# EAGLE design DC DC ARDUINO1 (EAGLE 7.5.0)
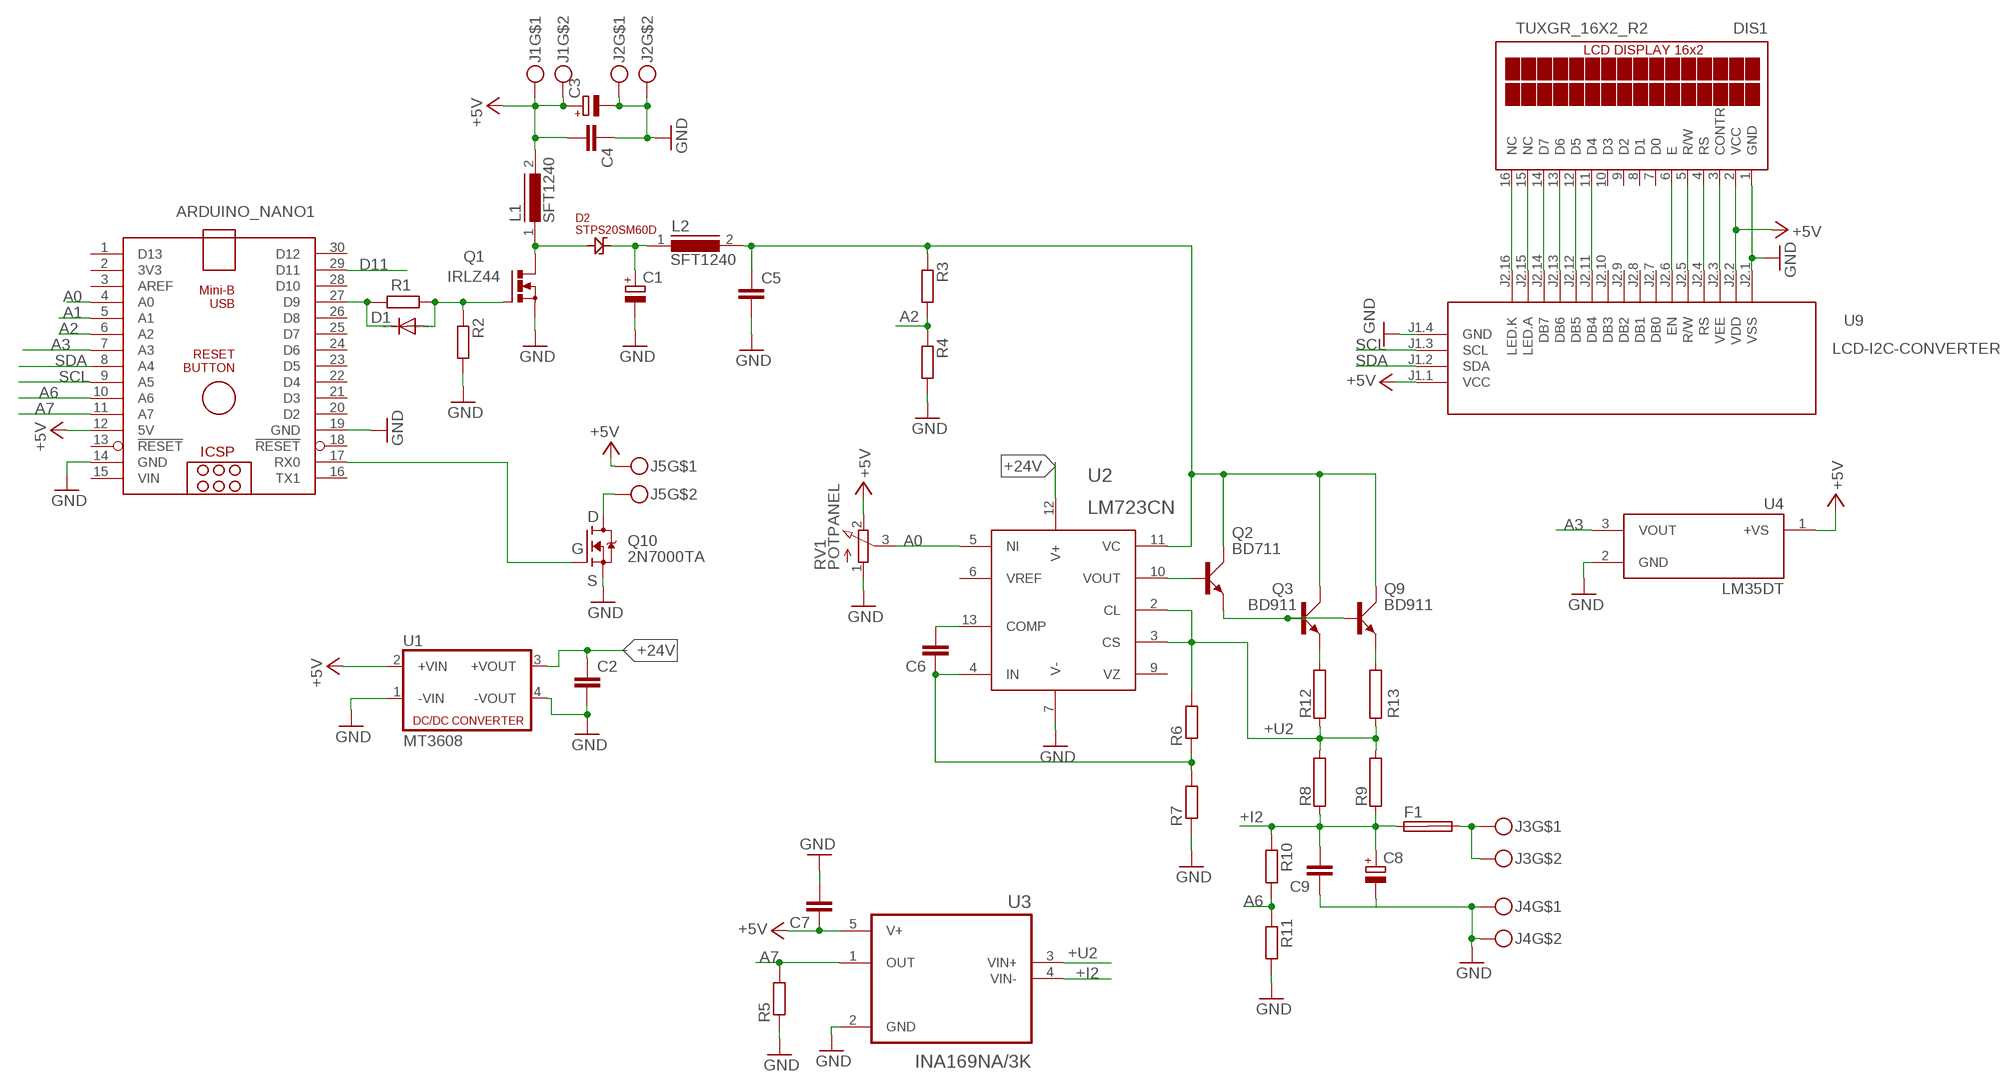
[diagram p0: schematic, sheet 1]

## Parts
ARDUINO_NANO1  ARDUINO_NANO  [ARDUINO_NANO]
C1  CPOL-EUE7.5-18  [E7,5-18]
C2  C-EU050-030X075  [C050-030X075]
C3  CPOL-EUE7.5-18  [E7,5-18]
C4  C-EU050-030X075  [C050-030X075]
C5  C-EU050-030X075  [C050-030X075]
C6  C-EU050-030X075  [C050-030X075]
C7  C-EU050-030X075  [C050-030X075]
C8  CPOL-EUE7.5-18  [E7,5-18]
C9  C-EU050-030X075  [C050-030X075]
D1  1N4148DO35-10  [DO35-10]
D2  STPS20SM60D  [TO-220-2]
DIS1  TUXGR_16X2_R2  [TUXGR_16X2_R2]
F1  SHK20L  [SHK20L]
J1  MKDSN1,5-2-5,08  [MKDSN1,5-2-5,08]
J2  MKDSN1,5-2-5,08  [MKDSN1,5-2-5,08]
J3  MKDSN1,5-2-5,08  [MKDSN1,5-2-5,08]
J4  MKDSN1,5-2-5,08  [MKDSN1,5-2-5,08]
J5  MKDSN1,5-2-5,08  [MKDSN1,5-2-5,08]
L1  SFT1240  [SFT1240]
L2  SFT1240  [SFT1240]
Q1  IRLZ44  IRF512  [TO220BV]
Q2  BD711  MJE3055  [TO220AV]
Q3  BD911  MJE3055  [TO220AV]
Q9  BD911  MJE3055  [TO220AV]
Q10  2N7000TA  [TO-92]
R1  R-EU_  [0204_6]
R2  R-EU_  [0204_6]
R3  R-EU_  [0204_6]
R4  R-EU_  [0204_6]
R5  R-EU_  [0204_6]
R6  R-EU_  [0204_6]
R7  R-EU_  [0204_6]
R8  RCA4050  [CA4050]
R9  RCA4050  [CA4050]
R10  R-EU_  [0204_6]
R11  R-EU_  [0204_6]
R12  RCA4050  [CA4050]
R13  RCA4050  [CA4050]
RV1  POTPANEL  [POTPANELP231]
U1  MT3608  [MT3608]
U2  LM723CN  [DIP14]
U3  INA169NA/3K  [SOT95P280X145-5N]
U4  LM35DT  [TO254P1016X457X1955-3]
U9  LCD-I2C-CONVERTER  [LCD-I2C-CONVERTER]

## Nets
+5V: ARDUINO_NANO1.12(5V) C3.+ C4.2 C7.1 DIS1.2(VCC) J1.1 J1.2 J5.1 L1.2 RV1.2(E) U1.2(+VIN) U3.5(V+) U4.1(+VS) U9.J1.1(VCC) U9.J2.2(VDD)
+24V: C2.1 U1.3(+VOUT) U2.12(V+)
+I2: C8.+ C9.2 F1.1A R8.1 R9.1 R10.1 U3.4(VIN-)
+U2: R6.2 R8.2 R9.2 R12.1 R13.1 U2.2(CL) U2.3(CS) U3.3(VIN+)
A0: ARDUINO_NANO1.4(A0) RV1.3(S) U2.5(NI)
A1: ARDUINO_NANO1.5(A1)
A2: ARDUINO_NANO1.6(A2) R3.2 R4.1
A3: ARDUINO_NANO1.7(A3) U4.3(VOUT)
A6: ARDUINO_NANO1.10(A6) R10.2 R11.1
A7: ARDUINO_NANO1.11(A7) R5.2 U3.1(OUT)
D11: ARDUINO_NANO1.29(D11)
GND: ARDUINO_NANO1.14(GND) ARDUINO_NANO1.19(GND) C1.- C2.2 C3.- C4.1 C5.2 C7.2 C8.- C9.1 DIS1.1(GND) J2.1 J2.2 J4.1 J4.2 Q1.S Q10.1(S) R2.2 R4.2 R5.1 R7.1 R11.2 RV1.1(A) U1.1(-VIN) U1.4(-VOUT) U2.7(V-) U3.2(GND) U4.2(GND) U9.J1.4(GND) U9.J2.1(VSS)
N$1: Q3.E R12.2
N$2: Q9.E R13.2
N$4: F1.2A J3.1 J3.2
N$5: ARDUINO_NANO1.17(RX0) Q10.2(G)
N$6: D1.A Q1.G R1.1 R2.1
N$7: ARDUINO_NANO1.27(D9) D1.C R1.2
N$8: D2.3(A) L1.1 Q1.D
N$9: J5.2 Q10.3(D)
N$10: C5.1 L2.2 Q2.C Q3.C Q9.C R3.1 U2.11(VC)
N$11: C1.+ D2.1(K) L2.1
N$23: C6.2 U2.13(COMP)
N$24: Q2.E Q3.B Q9.B
N$26: C6.1 R6.1 R7.2 U2.4(IN)
N$27: Q2.B U2.10(VOUT)
N$31: DIS1.3(CONTR) U9.J2.3(VEE)
N$32: DIS1.4(RS) U9.J2.4(RS)
N$33: DIS1.5(R/W) U9.J2.5(R/W)
N$34: DIS1.6(E) U9.J2.6(EN)
N$35: DIS1.14(D7) U9.J2.14(DB7)
N$36: DIS1.13(D6) U9.J2.13(DB6)
N$37: DIS1.12(D5) U9.J2.12(DB5)
N$38: DIS1.11(D4) U9.J2.11(DB4)
N$39: DIS1.16(NC) U9.J2.16(LED.K)
N$40: DIS1.15(NC) U9.J2.15(LED.A)
SCL: ARDUINO_NANO1.9(A5) U9.J1.3(SCL)
SDA: ARDUINO_NANO1.8(A4) U9.J1.2(SDA)
Unconnected: ARDUINO_NANO1.1(D13) ARDUINO_NANO1.2(3V3) ARDUINO_NANO1.3(AREF) ARDUINO_NANO1.13(!RESET) ARDUINO_NANO1.16(TX1) ARDUINO_NANO1.18(!RESET) ARDUINO_NANO1.20(D2) ARDUINO_NANO1.21(D3) ARDUINO_NANO1.22(D4) ARDUINO_NANO1.23(D5) ARDUINO_NANO1.24(D6) ARDUINO_NANO1.25(D7) ARDUINO_NANO1.26(D8) ARDUINO_NANO1.28(D10) ARDUINO_NANO1.30(D12) DIS1.7(D0) DIS1.8(D1) DIS1.9(D2) DIS1.10(D3) F1.1B F1.2B U2.6(VREF) U2.9(VZ) U9.J2.7(DB0) U9.J2.8(DB1) U9.J2.9(DB2) U9.J2.10(DB3)

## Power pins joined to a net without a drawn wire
VIN: ARDUINO_NANO1.15(VIN)

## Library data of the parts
ARDUINO_NANO1 = ArduinoNanoV30:ARDUINO_NANO: Arduino Nano V3.0 Overview: The Arduino Nano is a small, complete, and breadboard-friendly board based on the ATmega328 (Arduino Nano 3.x) or ATmega168 (Arduino Nano 2.x). It has more or less the same functionality of the Arduino Duemilanove, but in a different package. It lacks only a DC power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
C1 C3 C8 = rcl:CPOL-EU: POLARIZED CAPACITOR, European symbol
C2 C4-C7 C9 = rcl:C-EU: CAPACITOR, European symbol
D1 = diode:1N4148: DIODE
D2 = STPS20SM60D:STPS20SM60D: Diode Schottky 60V 20A Through Hole TO-220AC Check availability; AVAILABILITY: In Stock; CHECK_PRICES: https://www.snapeda.com/parts/STPS20SM60D/STMicroelectronics/view-part/?ref=eda; DESCRIPTION: Diode Schottky 60 V 20A Through Hole TO-220AC; MF: STMicroelectronics; MP: STPS20SM60D; PACKAGE: TO-220 STMicroelectronics; PRICE: None; PURCHASE-URL: https://www.snapeda.com/api/url_track_click_mouser/?unipart_id=727029&manufacturer=STMicroelectronics&part_name=STPS20SM60D&search_term=shottky diode 20a to-220; SNAPEDA_LINK: https://www.snapeda.com/parts/STPS20SM60D/STMicroelectronics/view-part/?ref=snap
DIS1 = display-lcd:TUXGR_16X2_R2: Tuxgraphics LCD display 16x2 characters reflective, without background light Source: tuxgr_12x2_r2.pdf; OC_FARNELL: unknown; OC_NEWARK: unknown
F1 = fuse:SHK20L: FUSE HOLDER 5 x 20 mm, SH contact, SHH1 Schukat, E1073 Buerklin; OC_FARNELL: unknown; OC_NEWARK: unknown
J1-J5 = con-phoenix-508:MKDSN1,5-2-5,08
L1 L2 = inductors:SFT1240: INDUCTOR
Q1 = transistor-power:IRF512: N-CHANNEL MOS FET
Q2 Q3 Q9 = transistor-power:MJE3055: NPN TRANSISTOR
Q10 = 2N7000TA:2N7000TA: http://www.mouser.com/ds/2/149/2N7000TA-347571.pdf Check availability; AVAILABILITY: In Stock; CHECK_PRICES: https://www.snapeda.com/parts/2N7000-TA/Onsemi/view-part/?ref=eda; DESCRIPTION: N-Channel 60 V 200mA (Tc) 400mW (Ta) Through Hole TO-92-3; MF: ON Semiconductor; MP: 2N7000-TA; PACKAGE: E-PKG AXIAL-LEADED-2 ON Semiconductor; PRICE: None; SNAPEDA_LINK: https://www.snapeda.com/parts/2N7000-TA/Onsemi/view-part/?ref=snap
R1-R7 R10 R11 = rcl:R-EU_: RESISTOR, European symbol
R8 R9 R12 R13 = resistor-power:R: Power Resitor; OC_FARNELL: unknown; OC_NEWARK: unknown
RV1 = pot:POTPANEL
U1 = dc-dc-converter:MT3608: DC DC Up Converter
U2 = v-reg:LM723CN: 150mA out, Voltage Regulator
U3 = INA169NA_3K:INA169NA/3K: Check availability; AVAILABILITY: In Stock; CHECK_PRICES: https://www.snapeda.com/parts/INA169NA/3K/Texas+Instruments/view-part/?ref=eda; DESCRIPTION: 2.7 to 60V, 440kHz Variable gain current sense amplifier; MF: Texas Instruments; MP: INA169NA/3K; PACKAGE: SOT-23-5 Texas Instruments; PRICE: None; PURCHASE-URL: https://pricing.snapeda.com/search?q=INA169NA/3K&ref=eda; SNAPEDA_LINK: https://www.snapeda.com/parts/INA169NA/3K/Texas+Instruments/view-part/?ref=snap
U4 = LM35DT-H:LM35DT: Check availability; AVAILABILITY: In Stock; CHECK_PRICES: https://www.snapeda.com/parts/LM35DT/Texas+Instruments/view-part/?ref=eda; DESCRIPTION: ±0.5°C 4V-30V, Temperature sensor with analog output 3-TO-220 0 to 100; MF: Texas Instruments; MP: LM35DT; PACKAGE: TO-220-3 Texas Instruments; PRICE: None; SNAPEDA_LINK: https://www.snapeda.com/parts/LM35DT/Texas+Instruments/view-part/?ref=snap
U9 = diy-modules:LCD-I2C-CONVERTER: I2C Bus to 4-Bit Parallel LCD Interface with LED backlight driver

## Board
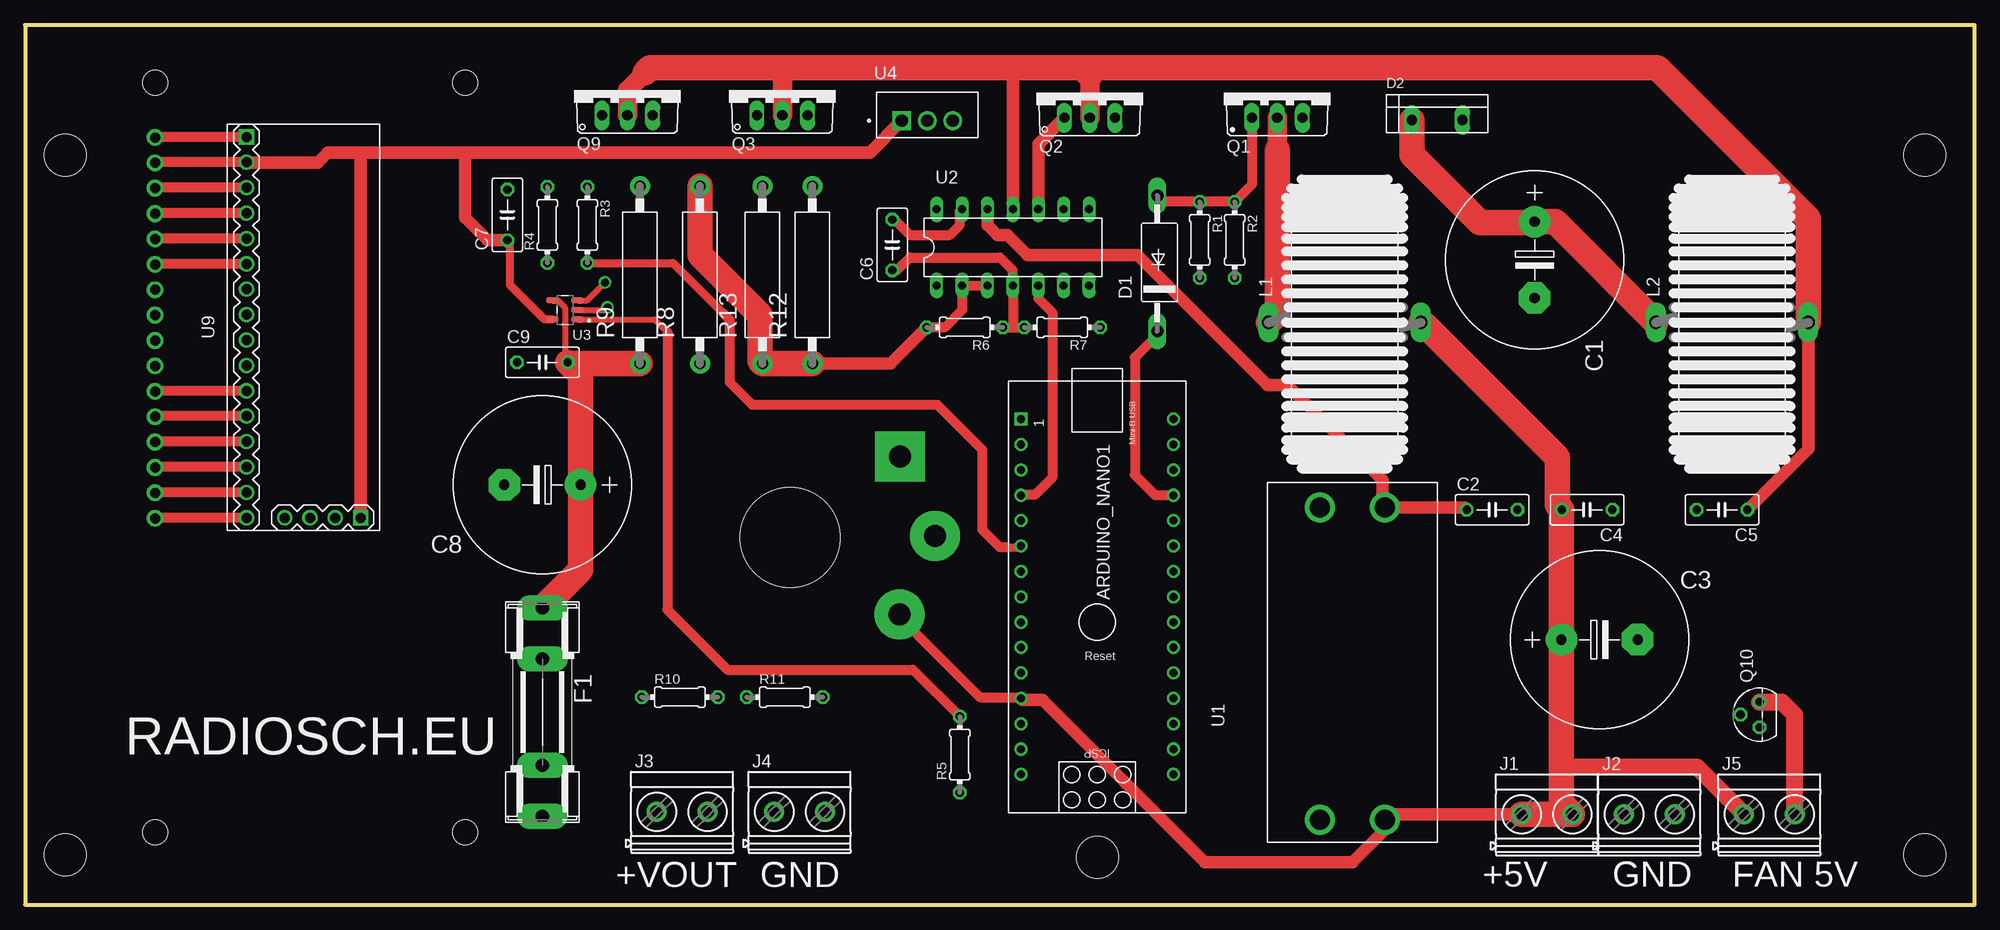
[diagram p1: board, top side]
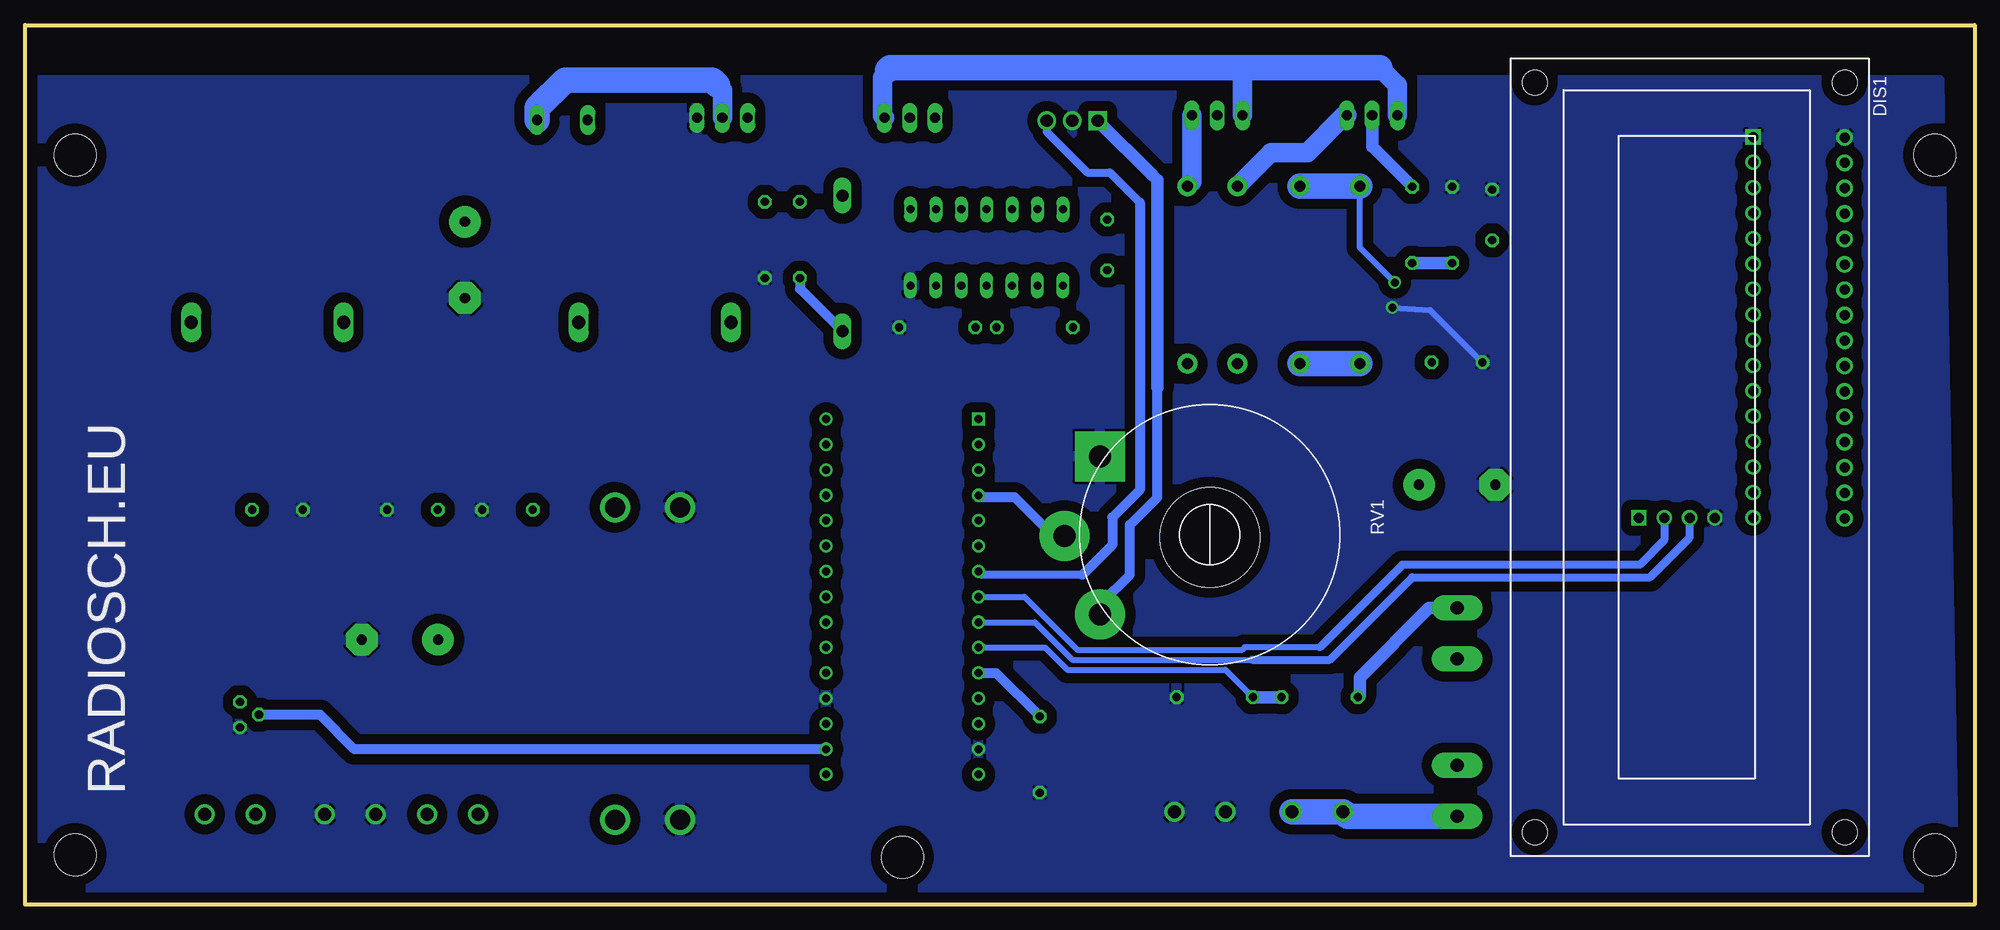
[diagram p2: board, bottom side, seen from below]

Size 195 x 88 mm. Coordinates in mm from the lower left corner, seen from the top.
Outline: 0,0 195,0 195,88 0,88 0,0
Copper layers (1*16): Top 0.035mm / dielectric 1.5mm / Bottom 0.035mm
Design rules "default": minimum track width 10mil, minimum drill 24mil, track to track 8mil, track to pad 8mil, pad to pad 8mil, via to via 8mil, smd to smd 8mil, copper to edge 40mil, drill to drill 8mil, minimum pad ring 10mil, minimum via ring 8mil, stop-mask expansion 4mil, vias tented up to drill 0mil, thermal gap 10mil
Holes 4.2 mm at 4,75 107.25,4.75 190,75 190,5 4,5
Holes 10 mm at 76.5,36.75

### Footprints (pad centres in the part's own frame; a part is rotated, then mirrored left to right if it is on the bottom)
ARDUINO_NANO = drill 0.8 square: 1 -20.32,-7.62 | drill 0.8: 2 -17.78,-7.62; 3 -15.24,-7.62; 4 -12.7,-7.62; 5 -10.16,-7.62; 6 -7.62,-7.62; 7 -5.08,-7.62; 8 -2.54,-7.62; 9 0,-7.62; 10 2.54,-7.62; 11 5.08,-7.62; 12 7.62,-7.62; 13 10.16,-7.62; 14 12.7,-7.62; 15 15.24,-7.62; 16 15.24,7.62; 17 12.7,7.62; 18 10.16,7.62; 19 7.62,7.62; 20 5.08,7.62; 21 2.54,7.62; 22 0,7.62; 23 -2.54,7.62; 24 -5.08,7.62; 25 -7.62,7.62; 26 -10.16,7.62; 27 -12.7,7.62; 28 -15.24,7.62; 29 -17.78,7.62; 30 -20.32,7.62
E7,5-18 = drill 1.016 pad 3.15: + -3.81,0 | drill 1.016 pad 3.15 octagon: - 3.81,0
C050-030X075 = drill 0.813 octagon: 1 -2.54,0; 2 2.54,0
DO35-10 = drill 1.2 long: A 8.18,0; C -5.38,0
TO-220-2 = drill 1.016 long: 1 -2.54,0; 3 2.54,0
TUXGR_16X2_R2 = drill 1 pad 1.676: 1 -32,15.5; 2 -29.46,15.5; 3 -26.92,15.5; 4 -24.38,15.5; 5 -21.84,15.5; 6 -19.3,15.5; 7 -16.76,15.5; 8 -14.22,15.5; 9 -11.68,15.5; 10 -9.14,15.5; 11 -6.6,15.5; 12 -4.06,15.5; 13 -1.52,15.5; 14 1.02,15.5; 15 3.56,15.5; 16 6.1,15.5 | hole 2.5: -37.5,-15.5; 37.5,-15.5; -37.5,15.5; 37.5,15.5
SHK20L = drill 1.321 pad 2.54 long: 1A -10.414,0; 1B -5.334,0; 2A 10.414,0; 2B 5.334,0
MKDSN1,5-2-5,08 = drill 1.3 pad 2: 1 -2.561,0.025; 2 2.519,0.025
SFT1240 = drill 1.321 long: 1 -7.62,0; 2 7.62,0
TO220BV = drill 1.016 long: D 0,-2.54; G -2.54,-2.54; S 2.54,-2.54
TO220AV = drill 1.016 long: B -2.54,-2.54; C 0,-2.54; E 2.54,-2.54
TO-92 = drill 0.813 octagon: 1 -1.27,0; 2 0,1.905; 3 1.27,0
0204_6 = drill 0.813 octagon: 1 -3.81,0; 2 3.81,0
CA4050 = drill 1.1 pad 2: 1 -8.89,0; 2 8.89,0
POTPANELP231 = drill 2.2 pad 5 square: 1 -7.85,-11 | drill 2.2 pad 5: 2 7.97,-10.96; 3 0.11,-14.54
MT3608 = drill 2: 1 2.25,11.75; 2 2.25,5.25; 3 33.5,5.25; 4 33.5,11.75
DIP14 = drill 0.813 long: 1 -3.81,-3.81; 2 -1.27,-3.81; 3 1.27,-3.81; 4 3.81,-3.81; 5 6.35,-3.81; 6 8.89,-3.81; 7 11.43,-3.81; 8 11.43,3.81; 9 8.89,3.81; 10 6.35,3.81; 11 3.81,3.81; 12 1.27,3.81; 13 -1.27,3.81; 14 -3.81,3.81
SOT95P280X145-5N = smd 1.21 x 0.59: 1 -1.255,0.95; 2 -1.255,0; 3 -1.255,-0.95; 4 1.255,-0.95; 5 1.255,0.95
TO254P1016X457X1955-3 = drill 1.24 square: 1 -2.54,-0.573 | drill 1.24: 2 0,-0.573; 3 2.54,-0.573
LCD-I2C-CONVERTER = drill 1 square: J1.1 -19.05,-5.08; J2.1 19.05,6.35 | drill 1: J1.2 -19.05,-2.54; J1.3 -19.05,0; J1.4 -19.05,2.54; J2.2 16.51,6.35; J2.3 13.97,6.35; J2.4 11.43,6.35; J2.5 8.89,6.35; J2.6 6.35,6.35; J2.7 3.81,6.35; J2.8 1.27,6.35; J2.9 -1.27,6.35; J2.10 -3.81,6.35; J2.11 -6.35,6.35; J2.12 -8.89,6.35; J2.13 -11.43,6.35; J2.14 -13.97,6.35; J2.15 -16.51,6.35; J2.16 -19.05,6.35

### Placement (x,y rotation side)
ARDUINO_NANO1  107.25,28.25 270 top
C1  151,64.5 270 top
C2  146.75,39.5 0 top
C3  157.5,26.5 0 top
C4  156.25,39.5 180 top
C5  169.75,39.5 180 top
C6  86.75,66 90 top
C7  48.25,69 90 top
C8  51.75,42 180 top
C9  51.75,54.25 0 top
D1  113.25,62.75 90 top
D2  141.25,78.5 0 top
DIS1  28.5,44.75 270 bottom
F1  51.75,19.25 270 top
J1  152.25,9 0 top
J2  162.5,9 0 top
J3  65.75,9.25 0 top
J4  77.5,9.25 0 top
J5  174.5,9 0 top
L1  132,58.25 0 top
L2  170.75,58.25 0 top
Q1  125.25,81.25 0 top
Q2  106.5,81.25 0 top
Q3  75.75,81.5 0 top
Q9  60.25,81.5 0 top
Q10  173.5,19 90 top
R1  117.5,66.5 270 top
R2  121,66.5 270 top
R3  56.25,68 270 top
R4  52.25,68 90 top
R5  93.5,15 90 top
R6  94,57.75 180 top
R7  103.75,57.75 180 top
R8  67.5,63 90 top
R9  61.5,63 90 top
R10  65.5,20.75 0 top
R11  76,20.75 0 top
R12  78.75,63 90 top
R13  73.75,63 90 top
RV1  76.5,37 270 bottom
U1  141.25,6.25 90 top
U2  95,65.75 0 top
U3  54,59.5 180 top
U4  90.25,79 0 top
U9  28.5,57.75 90 top

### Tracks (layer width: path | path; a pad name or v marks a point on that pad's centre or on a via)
+5V
  Top 0.813: U3.5 51.95,58.55 48.5,62 48.5,66.21 C7.1
  Top 1.016: U9.J2.2 13.05,74.26 DIS1.2 | RV1.2 87.46,28.79 95.5,20.75 99.51,20.75 ARDUINO_NANO1.12
  Top 1.27: U4.1 87.68,78.43 84.5,75.25 43.75,75.25 | 43.75,75.25 33.75,75.25 | 33.75,75.25 30.25,75.25 29.25,74.25 U9.J2.2 | C7.1 46.29,66.46 44,68.75 44,75 43.75,75.25 | U9.J1.1 33.58,75.08 33.75,75.25 | ARDUINO_NANO1.12 99.76,20.5 101.75,20.5 118,4.25 132.75,4.25 136,7.5 U1.2 136.53,9.03 J1.1
  Top 1.676: J5.1 171.94,9.06 167.25,13.75 153.69,13.75
  Top 2.54: L1.2 139.75,58.25 153.25,44.75 153.25,39.96 153.69,39.52 | 153.69,39.52 C4.2 | 153.69,39.52 C3.+ 153.69,13.75 153.69,10.1 J1.2 J1.1
  Bottom 1.016: 81.75,51.75 81.75,40.75 84.5,38 84.5,33 87.22,30.28 87.22,29.27 RV1.2
  Bottom 1.27: U4.1 82.25,72.97 82.22,72.97 81.75,72.5 81.75,51.75
+24V
  Top 1.27: U2.12 96.27,67.98 97.25,67 98.25,67 100.25,65 111.25,65 124.25,52 126.25,52 135.75,42.5 135.75,40 U1.3 143.96,39.75 C2.1
+I2
  Top 0.61: U3.4 53.3,60.45 54,59.75 54,54.54 C9.2
  Top 2.54: R9.1 54.43,54.11 C9.2 55.56,52.98 C8.+ 55.56,33.47 F1.1A
  Bottom 1.27: F1.1A 54.59,29.66 61.5,22.75 61.5,20.94 R10.1
  Bottom 2.54: R9.1 R8.1
+U2  (via drill 0.8)
  Top 0.61: U3.3 56.2,60.45 v58,62.25
  Top 1.016: R6.2 92,57.75 93.73,59.48 U2.2 U2.3
  Top 1.27: R12.1 86.55,54.11 R6.2
  Top 2.54: R8.2 67.5,65 73.5,59 73.5,54.36 R13.1 R12.1
  Bottom 0.61: v58,62.25 61.5,65.75 R9.2
  Bottom 2.54: R9.2 R8.2
A0
  Top 1.016: U2.5 101.35,60.65 102.75,59.25 102.75,42.75 101,41 99.68,41 ARDUINO_NANO1.4
  Bottom 1.016: RV1.3 92.14,36.89 96,40.75 99.43,40.75 ARDUINO_NANO1.4
A2
  Top 0.813: R3.2 64.81,64.19 69.88,59.12 | 98.25,35.75 99.51,35.75 ARDUINO_NANO1.6
  Top 1.016: 69.88,59.12 70.5,58.5 70.5,52.25 72.75,50 91.25,50 95.75,45.5 95.75,37.5 97.5,35.75 98.25,35.75
  Bottom 1.27: R3.2 R4.1
A3
  Bottom 0.813: U4.3 92.79,77.29 88.75,73.25 86.5,73.25 83.5,70.25 | 89.25,33 99.3,33 ARDUINO_NANO1.7
  Bottom 1.016: 83.5,70.25 83.5,41.5 86.25,38.75 86.25,36 89.25,33
A6
  Bottom 0.61: ARDUINO_NANO1.10 92.96,25.71 90.75,23.5 74.94,23.5 R11.1
  Bottom 1.27: R10.2 R11.1
A7
  Top 0.61: U3.1 62.95,58.55 64.25,57.25
  Top 1.016: 64.25,57.25 64.25,29.5 70.25,23.5 88.81,23.5 R5.2
  Bottom 1.016: ARDUINO_NANO1.11 97.86,23.17 R5.2
GND  (via drill 0.8)
  Top 0.61: U3.2 58,59.5 v58.25,59.75
  Top 1.016: U9.J2.1 13.05,76.8 DIS1.1
  Bottom 0.61: v58.25,59.75 54.46,59.5 C9.1
  pour Bottom (isolate 1.016): 3.5,82.5 197,82.5 195.5,1.5 2,1.5
N$1
  Bottom 1.93: Q3.E 78.29,72.35 R12.2
N$2
  Bottom 1.93: Q9.E 63.04,78.96 66.75,75.25 70.39,75.25 R13.2
N$4
  Bottom 2.54: F1.2A 62.75,8.84 J3.1 J3.2
N$5
  Bottom 1.016: ARDUINO_NANO1.17 162.05,15.55 165.5,19 Q10.2
N$6
  Top 1.016: Q1.G 122.71,72.02 R2.1 R1.1 113.87,70.31 D1.A
N$7
  Top 1.016: D1.C 113.25,57 111,54.75 111,43 113,41 114.82,41 ARDUINO_NANO1.27
  Bottom 1.016: R1.2 117.5,61.62 D1.C
N$8
  Top 1.93: Q1.D 125.25,75.5
  Top 2.54: 125.25,75.5 125.25,59.12 L1.1
  Bottom 1.93: Q1.D 125.25,81.5 125.75,82
  Bottom 2.54: D2.3 143.79,79.71 141,82.5 126.25,82.5 125.75,82
N$9
  Top 1.676: J5.2 177.02,18.98 175.75,20.25 173.52,20.25 Q10.3
N$10
  Top 1.27: L2.2 178.37,45.58 C5.1 | U2.11 98.81,83.31 99.25,83.75
  Top 1.93: Q9.C 60.25,81.5 62,83.25 | 106.5,83 Q2.C | Q3.C 75.75,83.25 75.25,83.75
  Top 2.54: 62,83.25 62.5,83.75 75.25,83.75 99.25,83.75 105.75,83.75 | 105.75,83.75 106.5,83 | L2.2 178.37,68.63 163.25,83.75 105.75,83.75
  Bottom 1.27: Q9.C 60.25,75.81 R3.1
N$11
  Top 2.54: D2.1 138.71,75.04 145.5,68.25 150.94,68.25 C1.+ 153.07,68.31 L2.1
N$23
  Top 1.016: C6.2 86.96,68.54 88.5,67 92.5,67 93.5,68 93.5,69.33 U2.13
N$24
  Bottom 1.93: Q9.B 57.71,81.96 59.5,83.75 | 108.75,83.5 108.75,83.25 109.25,82.75 109.25,78.92 Q2.E | Q3.B 73.21,83.71 73.25,83.75
  Bottom 2.54: 59.5,83.75 73.25,83.75 108.5,83.75 108.75,83.5
N$26
  Top 1.016: C6.1 87.21,63.46 88.5,64.75 97.5,64.75 98.75,63.5 98.75,62 U2.4 98.81,57.94 99,57.75 | R6.1 99,57.75 | 99,57.75 R7.2
N$27
  Top 1.27: U2.10 101.35,76.1 Q2.B
N$31
  Top 1.016: U9.J2.3 13.05,71.72 DIS1.3
N$32
  Top 1.016: U9.J2.4 13.05,69.18 DIS1.4
N$33
  Top 1.016: U9.J2.5 13.05,66.64 DIS1.5
N$34
  Top 1.016: U9.J2.6 13.05,64.1 DIS1.6
N$35
  Top 1.016: U9.J2.14 13.05,43.78 DIS1.14
N$36
  Top 1.016: U9.J2.13 13.05,46.32 DIS1.13
N$37
  Top 1.016: U9.J2.12 13.05,48.86 DIS1.12
N$38
  Top 1.016: U9.J2.11 13.05,51.4 DIS1.11
N$39
  Top 1.016: U9.J2.16 13.05,38.7 DIS1.16
N$40
  Top 1.016: U9.J2.15 13.05,41.24 DIS1.15
SCL
  Bottom 0.61: ARDUINO_NANO1.9 94,28.25 90.25,24.5 72.25,24.5
  Bottom 0.813: 72.25,24.5 64.5,24.5 56.25,32.75 32.5,32.75 28.5,36.75 U9.J1.3
SDA
  Bottom 0.61: ARDUINO_NANO1.8 95.04,30.79 89.75,25.5 73.25,25.5 73,25.75 65.5,25.75
  Bottom 0.813: U9.J1.2 31.04,36.46 33.5,34 57.25,34 65.5,25.75

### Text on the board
tPlace: RADIOSCH.EU | +VOUT | GND | +5V | GND | FAN 5V
bPlace: RADIOSCH.EU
